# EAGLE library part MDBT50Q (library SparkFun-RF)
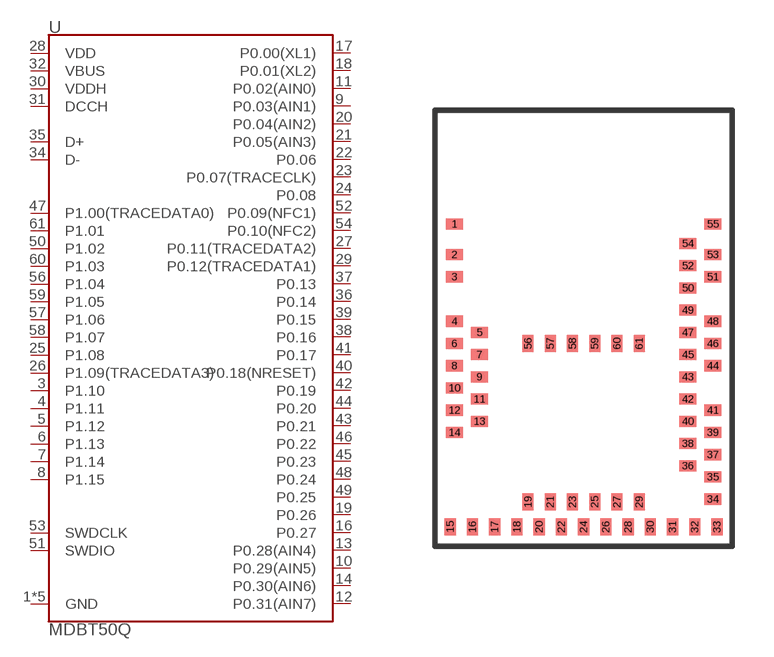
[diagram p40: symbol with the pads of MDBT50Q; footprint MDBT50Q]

Designator prefix U

## MDBT50Q (PROD_ID: IC-14109)  [MDBT50Q]
1  GND
2  GND
3  P1.10
4  P1.11
5  P1.12
6  P1.13
7  P1.14
8  P1.15
9  P0.03(AIN1)
10  P0.29(AIN5)
11  P0.02(AIN0)
12  P0.31(AIN7)
13  P0.28(AIN4)
14  P0.30(AIN6)
15  GND
16  P0.27
17  P0.00(XL1)
18  P0.01(XL2)
19  P0.26
20  P0.04(AIN2)
21  P0.05(AIN3)
22  P0.06
23  P0.07(TRACECLK)
24  P0.08
25  P1.08
26  P1.09(TRACEDATA3)
27  P0.11(TRACEDATA2)
28  VDD
29  P0.12(TRACEDATA1)
30  VDDH
31  DCCH
32  VBUS
33  GND
34  D-
35  D+
36  P0.14
37  P0.13
38  P0.16
39  P0.15
40  P0.18(NRESET)
41  P0.17
42  P0.19
43  P0.21
44  P0.20
45  P0.23
46  P0.22
47  P1.00(TRACEDATA0)
48  P0.24
49  P0.25
50  P1.02
51  SWDIO
52  P0.09(NFC1)
53  SWDCLK
54  P0.10(NFC2)
55  GND
56  P1.04
57  P1.06
58  P1.07
59  P1.05
60  P1.03
61  P1.01

## Footprint MDBT50Q (pad centres in mm)
smd 0.6 x 0.4: 1 -4.65,3.65; 2 -4.65,2.55; 3 -4.65,1.75; 4 -4.65,0.15; 5 -3.75,-0.25; 6 -4.65,-0.65; 7 -3.75,-1.05; 8 -4.65,-1.45; 9 -3.75,-1.85; 10 -4.65,-2.25; 11 -3.75,-2.65; 12 -4.65,-3.05; 13 -3.75,-3.45; 14 -4.65,-3.85; 34 4.65,-6.25; 35 4.65,-5.45; 36 3.75,-5.05; 37 4.65,-4.65; 38 3.75,-4.25; 39 4.65,-3.85; 40 3.75,-3.45; 41 4.65,-3.05; 42 3.75,-2.65; 43 3.75,-1.85; 44 4.65,-1.45; 45 3.75,-1.05; 46 4.65,-0.65; 47 3.75,-0.25; 48 4.65,0.15; 49 3.75,0.55; 50 3.75,1.35; 51 4.65,1.75; 52 3.75,2.15; 53 4.65,2.55; 54 3.75,2.95; 55 4.65,3.65
smd 0.4 x 0.6: 15 -4.8,-7.25; 16 -4,-7.25; 17 -3.2,-7.25; 18 -2.4,-7.25; 19 -2,-6.35; 20 -1.6,-7.25; 21 -1.2,-6.35; 22 -0.8,-7.25; 23 -0.4,-6.35; 24 0,-7.25; 25 0.4,-6.35; 26 0.8,-7.25; 27 1.2,-6.35; 28 1.6,-7.25; 29 2,-6.35; 30 2.4,-7.25; 31 3.2,-7.25; 32 4,-7.25; 33 4.8,-7.25; 56 -2,-0.65; 57 -1.2,-0.65; 58 -0.4,-0.65; 59 0.4,-0.65; 60 1.2,-0.65; 61 2,-0.65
